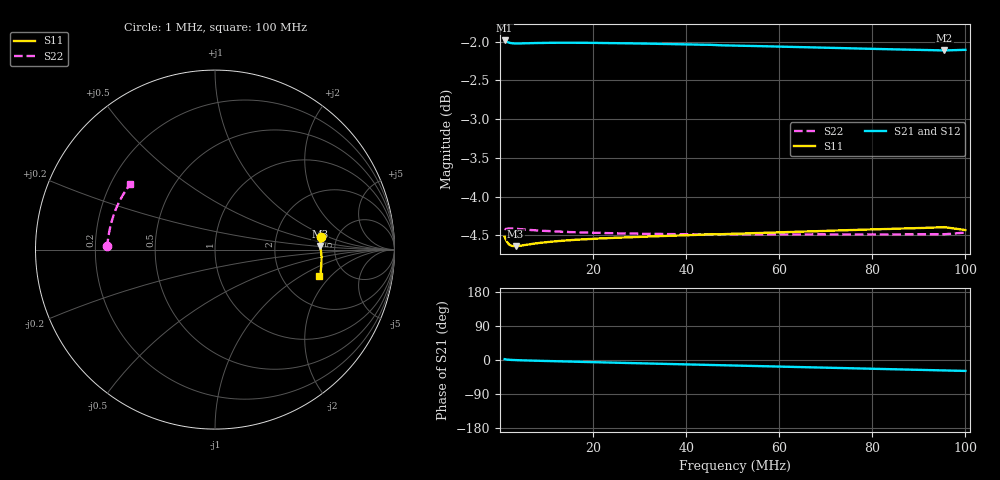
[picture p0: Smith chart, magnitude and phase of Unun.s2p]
! ListType=Log
!!Unun
# MHZ S RI R 50
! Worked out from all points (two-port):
!   100 points, 1 MHz to 100 MHz, reference 50 ohm
!   highest |S21| = -1.98 dB at 1 MHz (marker M1); lowest = -2.1 dB at 95.45 MHz (marker M2)
!   |S21| within 3 dB of the highest: start of sweep to end of sweep
!   lowest |S11| = -4.6 dB at 3.352 MHz (marker M3), VSWR 3.83, Z = 191 + j10.2 ohm
!   |S11| at or under -10 dB: nowhere
!   |S22| runs from -4.5 to -4.4 dB; largest |S21 - S12| = 0.0088
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1  0.5902 0.0701  0.7952 0.0311  0.7954 0.0313  -0.6009 0.0226
1.149757  0.59 0.0593  0.795 0.0252  0.7952 0.0253  -0.6009 0.0206
1.321941  0.5893 0.0501  0.7946 0.0199  0.7948 0.02  -0.6009 0.0191
1.519911  0.5884 0.0424  0.7941 0.0154  0.7943 0.0155  -0.6011 0.0181
1.747528  0.5875 0.0361  0.7935 0.0114  0.7938 0.0116  -0.6013 0.0176
2.009233  0.5867 0.0308  0.7931 0.00784  0.7933 0.00806  -0.6013 0.0175
2.31013  0.5862 0.0264  0.7928 0.00459  0.793 0.00482  -0.6014 0.0178
2.782559  0.5858 0.0216  0.7924 0.000489  0.7927 0.000769  -0.6013 0.0187
3.351603  0.5858 0.0175  0.7923 -0.00353  0.7925 -0.00323  -0.6011 0.0203
5.336699  0.587 0.00899  0.7923 -0.0147  0.7926 -0.0142  -0.6001 0.027
8.111308  0.5887 0.00166  0.7923 -0.0278  0.7927 -0.0272  -0.5988 0.0374
17.8865  0.5918 -0.0163  0.79 -0.0697  0.7908 -0.0684  -0.5934 0.0754
27.18588  0.593 -0.0311  0.7851 -0.1077  0.7865 -0.106  -0.5867 0.1116
34.30469  0.5934 -0.042  0.78 -0.1361  0.7819 -0.1343  -0.5804 0.1389
45.34879  0.5938 -0.0586  0.77 -0.1795  0.7728 -0.1778  -0.5684 0.1803
52.14008  0.5932 -0.0693  0.7623 -0.2055  0.7657 -0.2039  -0.56 0.2054
59.94843  0.5927 -0.0815  0.7527 -0.235  0.7566 -0.2338  -0.5489 0.2335
68.92612  0.5917 -0.0959  0.7403 -0.2684  0.7446 -0.2676  -0.5345 0.2648
79.24829  0.5901 -0.1129  0.7241 -0.3058  0.7288 -0.3059  -0.5158 0.2993
86.9749  0.5884 -0.126  0.7108 -0.3332  0.7157 -0.334  -0.5008 0.324
95.45485  0.5862 -0.1409  0.6951 -0.3628  0.6999 -0.3644  -0.483 0.3501
100  0.582 -0.1472  0.6876 -0.3783  0.695 -0.3832  -0.4744 0.3642
